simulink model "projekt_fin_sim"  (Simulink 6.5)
settings: Solver=ode45  StartTime=0.0  StopTime=10  FixedStep=0.01  RelTol=1e-3
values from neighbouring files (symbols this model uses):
  A = [dh1_h10 dh1_h20 0    [podklad.m]    (also in testx.m = [ -0.195 0.195; 0.195 -0.205]; kockaLQG.m = [0 1 0 0 0; kockaLQR.m = [0 1 0 0 0; kulicka_na_tyci_LQG_podklad.m = [0 0;1 0])
  B = [dh1_q0    [podklad.m]    (also in testx.m = [0.0047; 0]; kockaLQG.m = [0; kockaLQR.m = [0; kulicka_na_tyci_LQG_podklad.m = [7.14;0])
  C = [0 0 1]    [podklad.m]    (also in testx.m = [0 1]; kockaLQG.m = [1 0 0 0 0]; kockaLQR.m = [1 0 0 0 0]; kulicka_na_tyci_LQG_podklad.m = [0 1])
  D = 0    [podklad.m]    (also in testx.m = [0]; kockaLQG.m = [0]; kockaLQR.m = [0]; kulicka_na_tyci_LQG_podklad.m)
  Hsens = ss(sysic)    [podklad.m]
  Wsnois1 = 0.01    [podklad.m]
  Wsnois2 = 0.01    [podklad.m]
undefined symbols (not defined in the file or in its folder): KA, KB, KC, KD

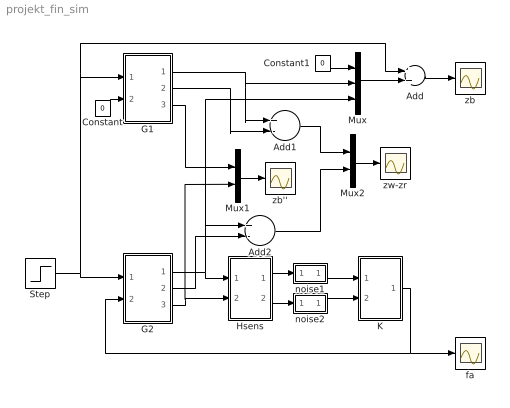
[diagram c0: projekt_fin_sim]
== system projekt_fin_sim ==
  Add : Sum  OutScaling=2^-10
  Add1 : Sum  Inputs=+-  OutScaling=2^-10
  Add2 : Sum  Inputs=+-  OutScaling=2^-10
  Constant : Constant  Value=0  OutDataType=sfix(16)  ConRadixGroup=Use specified scaling  OutScaling=2^0  SampleTime=inf  FramePeriod=inf
  Constant1 : Constant  Value=0  OutDataType=sfix(16)  ConRadixGroup=Use specified scaling  OutScaling=2^0  SampleTime=inf  FramePeriod=inf
  G1 : Subsystem
  G2 : Subsystem
  Hsens : Subsystem
  K : Subsystem
  Mux : Mux  Inputs=3
  Mux1 : Mux  Inputs=2
  Mux2 : Mux  Inputs=2
  Step : Step  Time=5  Before=0.1  After=0  SampleTime=0
  fa : Scope
  noise1 : Subsystem
  noise2 : Subsystem
  zb : Scope
  zb'' : Scope
  zw-zr : Scope
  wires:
  Step/1 -> G2/1(zr), Add/1, G1/1(zr)
  K/1(fa) -> fa/1, G2/2(fa)
  G2/3(zb'') -> Mux1/2, Hsens/2(zb'')
  Hsens/1(zr) -> noise1/1(in)
  Hsens/2(zb) -> noise2/1(in)
  noise2/1(out) -> K/2(zb)
  Constant/1 -> G1/2(fa)
  Add/1 -> zb/1
  G2/1(zb-zr) -> Hsens/1(zb-zr), Add2/1, Mux/3
  Mux1/1 -> zb''/1
  G1/3(zb'') -> Mux1/1
  noise1/1(out) -> K/1(zr)
  Mux/1 -> Add/2
  Mux2/1 -> zw-zr/1
  G1/1(zb-zr) -> Add1/1, Mux/2
  G1/2(zb-zw) -> Add1/2
  Add1/1 -> Mux2/1
  G2/2(zb-zw) -> Add2/2
  Add2/1 -> Mux2/2
  Constant1/1 -> Mux/1

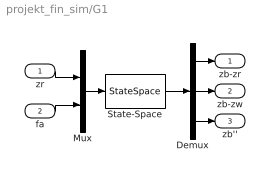
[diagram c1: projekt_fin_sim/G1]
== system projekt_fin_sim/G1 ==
  zr : Inport
  fa : Inport  Port=2
  Demux : Demux  Outputs=3
  Mux : Mux  Inputs=2
  State-Space : StateSpace  A=A  B=B  C=C  D=D
  zb-zr : Outport
  zb-zw : Outport  Port=2
  zb'' : Outport  Port=3
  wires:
  Demux/3 -> zb''/1
  fa/1 -> Mux/2
  Demux/2 -> zb-zw/1
  zr/1 -> Mux/1
  Demux/1 -> zb-zr/1
  State-Space/1 -> Demux/1
  Mux/1 -> State-Space/1

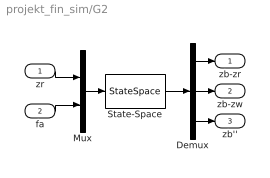
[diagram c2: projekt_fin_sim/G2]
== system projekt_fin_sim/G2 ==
  zr : Inport
  fa : Inport  Port=2
  Demux : Demux  Outputs=3
  Mux : Mux  Inputs=2
  State-Space : StateSpace  A=A  B=B  C=C  D=D
  zb-zr : Outport
  zb-zw : Outport  Port=2
  zb'' : Outport  Port=3
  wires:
  Mux/1 -> State-Space/1
  State-Space/1 -> Demux/1
  Demux/1 -> zb-zr/1
  zr/1 -> Mux/1
  Demux/2 -> zb-zw/1
  fa/1 -> Mux/2
  Demux/3 -> zb''/1

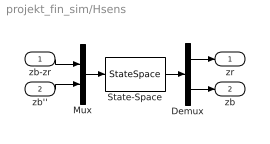
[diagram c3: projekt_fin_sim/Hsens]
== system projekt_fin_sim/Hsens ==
  zb-zr : Inport
  zb'' : Inport  Port=2
  Demux : Demux  Outputs=2
  Mux : Mux  Inputs=2
  State-Space : StateSpace  A=Hsens.a  B=Hsens.b  C=Hsens.c  D=Hsens.d
  zr : Outport
  zb : Outport  Port=2
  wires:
  Mux/1 -> State-Space/1
  State-Space/1 -> Demux/1
  Demux/1 -> zr/1
  zb-zr/1 -> Mux/1
  Demux/2 -> zb/1
  zb''/1 -> Mux/2

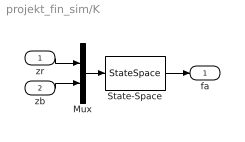
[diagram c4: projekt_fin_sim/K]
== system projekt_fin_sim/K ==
  zr : Inport
  zb : Inport  Port=2
  Mux : Mux  Inputs=2
  State-Space : StateSpace  A=KA  B=KB  C=KC  D=KD
  fa : Outport
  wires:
  Mux/1 -> State-Space/1
  zr/1 -> Mux/1
  State-Space/1 -> fa/1
  zb/1 -> Mux/2

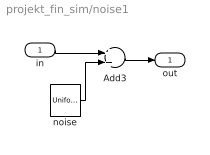
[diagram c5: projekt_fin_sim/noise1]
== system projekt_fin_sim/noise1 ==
  in : Inport
  Add3 : Sum  OutScaling=2^-10
  noise : UniformRandomNumber  Minimum=-Wsnois1  Maximum=Wsnois1  Seed=1  SampleTime=0
  out : Outport
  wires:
  noise/1 -> Add3/2
  in/1 -> Add3/1
  Add3/1 -> out/1

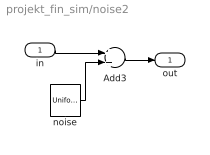
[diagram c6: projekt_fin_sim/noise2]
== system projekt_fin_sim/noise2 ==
  in : Inport
  Add3 : Sum  OutScaling=2^-10
  noise : UniformRandomNumber  Minimum=-Wsnois2  Maximum=Wsnois2  Seed=2  SampleTime=0
  out : Outport
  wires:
  Add3/1 -> out/1
  in/1 -> Add3/1
  noise/1 -> Add3/2
